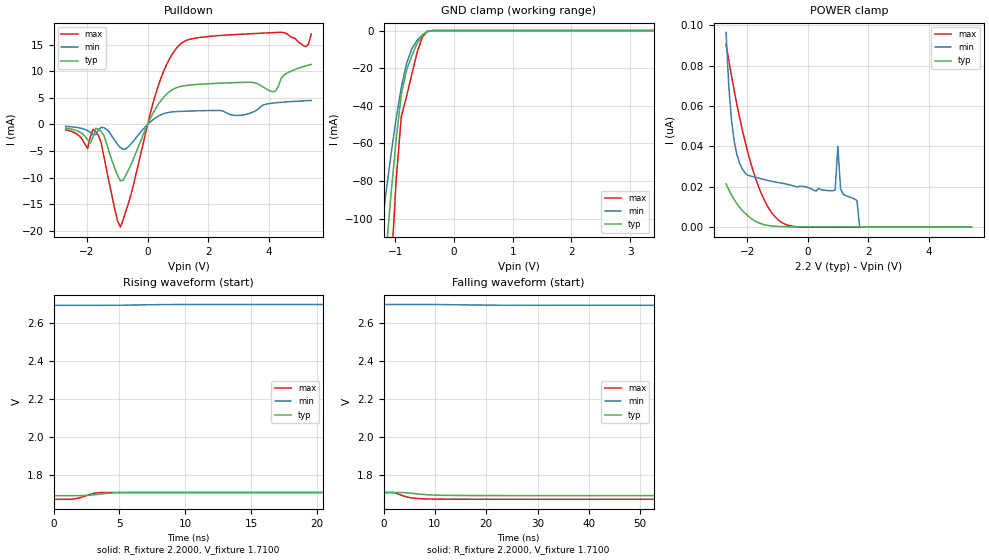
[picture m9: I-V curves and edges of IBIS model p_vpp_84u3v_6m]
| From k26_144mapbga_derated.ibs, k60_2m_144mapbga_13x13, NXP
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[Model] p_vpp_84u3v_6m
|   Model p_vpp_84u3v_6m
| Library cells for typ/min/max conditions are connected as defined below:
|  pad - External Pad
|  ipp_do - Core Input
|  ipp_obe - Output Buffer Enable
|  esd_boost - vdd_s_3v
|  esd_bus - vdd_s_3v
|  ipp_ina_hv - NC
|  ipp_ind - NC
|  ipp_ind_3v - NC
|  vdd_s_3v - vdd_s_3v
|  vdd_s_lv - vdd_s_lv
|  vpp1 - NC
|  vpp2 - NC
|  vss_bulk - vss_bulk
|  vss_s_lv - vss_s_lv
| All other pins connected to ground
Model_type I/O_open_drain
Polarity   Non-Inverting
Enable   Active-High
Vinl =   0.6600V
Vinh =   1.6500V
Vmeas =  1.1000V
Cref =   25.0000pF
Rref =   50.0000
Vref =   0.0V
C_comp   4.8667pF   4.6542pF   4.8793pF
[Temperature Range]   25.0000   0.1250k   -40.0000
[Voltage Range]   2.2000V   1.7100V   2.7000V
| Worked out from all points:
|   slope of the pulldown table from 0 to 0.33 V, typ, clamps not added: 92.3 ohm
|   GND clamp passes 1 mA (typ) near -0.48 V on its own axis
[Pulldown]
|Voltage   I(typ)   I(min)   I(max)
-2.7V     -714uA     -370uA     -1.022mA
-1.98V    -2.886mA   -1.171mA   -4.535mA
-1.8V     -2.349mA   -1.89mA    -905.1uA
-1.62V    -944.4uA   -1.003mA   -2.082mA
-900mV    -10.59mA   -4.35mA    -19.32mA
270mV     3.037mA    1.27mA     5.798mA
990mV     6.992mA    2.421mA    14.58mA
3.06V     7.892mA    1.716mA    16.95mA
4.14V     6.144mA    4.012mA    17.26mA
4.5V      9.306mA    4.201mA    17.27mA
5.22V     11.01mA    4.445mA    14.62mA
5.4V      11.26mA    4.493mA    16.99mA
[GND_clamp]
|Voltage   I(typ)   I(min)   I(max)
-2.7V     -9.648A    -10.17A    -9.383A
-1.26V    -157.5mA   -111mA     -244mA
-1.17V    -122.3mA   -88.72mA   -186.8mA
-1.08V    -89.05mA   -67.27mA   -131.6mA
-990mV    -58.85mA   -47.34mA   -81.19mA
-900mV    -34.22mA   -30.28mA   -45.91mA
-810mV    -21.08mA   -17.56mA   -35.14mA
-720mV    -13.41mA   -9.71mA    -23.25mA
-630mV    -6.896mA   -5.145mA   -11.62mA
-540mV    -2.367mA   -2.243mA   -3.384mA
-450mV    -342.3uA   -648.2uA   -233.3uA
5.4V      0A         0A         0A
[POWER_clamp]
|Voltage   I(typ)   I(min)   I(max)
-2.7V     21.49nA    96.52nA    90.61nA
-2.61V    18.58nA    69.78nA    82.65nA
-2.52V    15.97nA    52.98nA    74.95nA
-2.25V    9.724nA    31.58nA    54.12nA
-1.62V    2.117nA    24.28nA    19.79nA
-900mV    314.4pA    21.89nA    2.694nA
900mV     165.4pA    18.43nA    5.718pA
990mV     164.7pA    40.07nA    5.582pA
1.08V     161.5pA    18.89nA    5.263pA
1.62V     143.5pA    13.2nA     2.129pA
1.71V     127.5pA    0A         1.693pA
5.4V      0A         0A         0A
[Ramp]
| variable   typ   min   max
dV/dt_r  0.2277/1.4252n   21.1656m/1.2925n   0.4938/1.0139n
dV/dt_f  0.2274/4.5650n   21.1770m/4.8623n   0.4908/2.7053n
R_load = 50.0000
[Rising Waveform]
R_fixture= 2.2000
V_fixture= 1.7100
V_fixture_min= 2.7000
|time   V(typ)   V(min)   V(max)
0s        1.693V     2.696V     1.674V
1.21ns    1.693V     2.696V     1.674V
1.552ns   1.693V     2.696V     1.676V
1.908ns   1.694V     2.696V     1.681V
3.153ns   1.699V     2.696V     1.708V
3.7ns     1.703V     2.696V     1.71V
4.88ns    1.71V      2.696V     1.71V
5.818ns   1.71V      2.697V     1.71V
10.31ns   1.71V      2.7V       1.71V
350ns     1.71V      2.7V       1.71V
[Falling Waveform]
R_fixture= 2.2000
V_fixture= 1.7100
V_fixture_min= 2.7000
|time   V(typ)   V(min)   V(max)
0s        1.71V      2.7V       1.71V
2.069ns   1.71V      2.7V       1.709V
4.235ns   1.709V     2.7V       1.689V
4.844ns   1.708V     2.7V       1.685V
5.963ns   1.705V     2.7V       1.68V
8.498ns   1.698V     2.7V       1.676V
11.61ns   1.695V     2.7V       1.675V
21.51ns   1.694V     2.697V     1.675V
33.2ns    1.694V     2.696V     1.675V
350ns     1.694V     2.696V     1.674V
